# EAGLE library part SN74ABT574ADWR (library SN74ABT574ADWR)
Texas Instruments SN74ABT574ADWR, D Type Bus Interface Flip Flop, 3-State, 4.5 5.5 V, 20-Pin SOIC Source: Datasheet
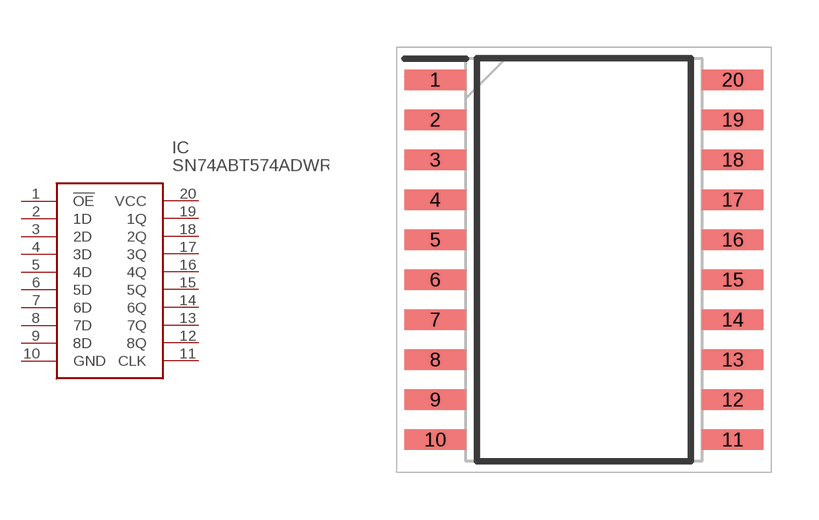
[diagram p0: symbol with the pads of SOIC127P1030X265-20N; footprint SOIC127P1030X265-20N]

Designator prefix IC

## SN74ABT574ADWR (Description: Texas Instruments SN74ABT574ADWR, D Type Bus Interface Flip Flop, 3-State, 4.5 5.5 V, 20-Pin SOIC; Height: 2.65mm; Manufacturer_Name: Texas Instruments; Manufacturer_Part_Number: SN74ABT574ADWR; Mouser_Part_Number: 595-SN74ABT574ADWR; Mouser_Price-Stock: https://www.mouser.co.uk/ProductDetail/Texas-Instruments/SN74ABT574ADWR?qs=nMmhAzRCgdCWNOUsuPi1DA%3D%3D)  [SOIC127P1030X265-20N]
1  !OE
2  1D
3  2D
4  3D
5  4D
6  5D
7  6D
8  7D
9  8D
10  GND
11  CLK
12  8Q
13  7Q
14  6Q
15  5Q
16  4Q
17  3Q
18  2Q
19  1Q
20  VCC

## Footprint SOIC127P1030X265-20N (pad centres in mm)
DW0020A HEIGHT 2.65_
smd 1.95 x 0.65: 1 -4.725,5.715; 2 -4.725,4.445; 3 -4.725,3.175; 4 -4.725,1.905; 5 -4.725,0.635; 6 -4.725,-0.635; 7 -4.725,-1.905; 8 -4.725,-3.175; 9 -4.725,-4.445; 10 -4.725,-5.715; 11 4.725,-5.715; 12 4.725,-4.445; 13 4.725,-3.175; 14 4.725,-1.905; 15 4.725,-0.635; 16 4.725,0.635; 17 4.725,1.905; 18 4.725,3.175; 19 4.725,4.445; 20 4.725,5.715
